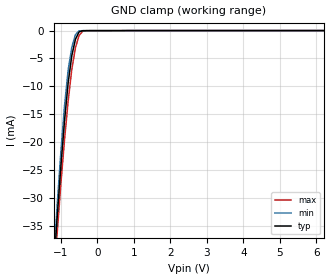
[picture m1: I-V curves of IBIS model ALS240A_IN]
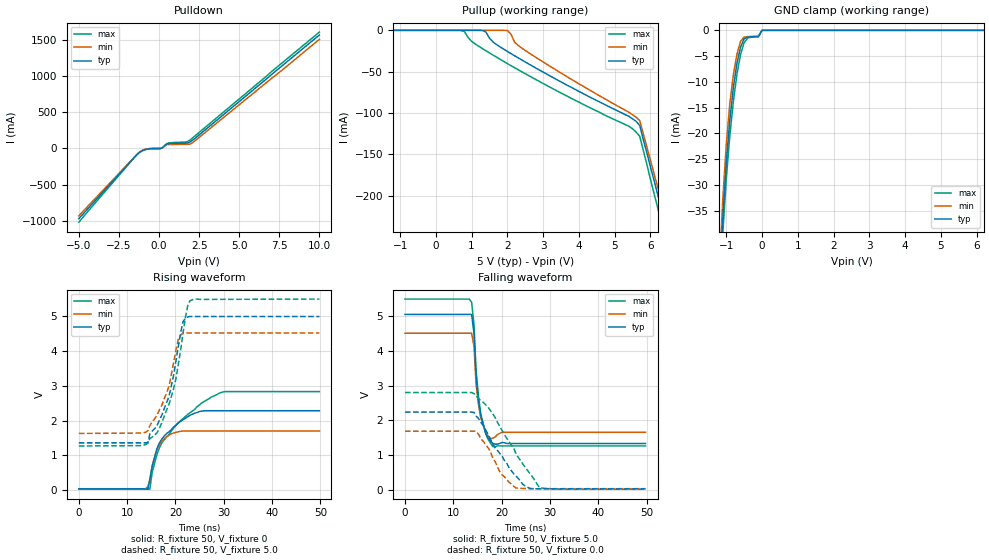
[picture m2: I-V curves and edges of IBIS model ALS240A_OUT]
| TEXAS INSTRUMENTS INCORPORATED
| Standard Linear and Logic Group
| IBIS Model of SN74ALS240A
| OCTAL BUFFERS/DRIVERS WITH 3-STATE OUTPUTS
| SOIC 20-pin (DW), SOP 20-pin (NS), SSOP 20-pin (DB), PDIP 20-pin (N) package
[IBIS Ver]   3.0
[Comment Char]  |_char
[File Name]   sn74als240a.ibs
[File Rev]   2.1
[Date]   Sept,22 2004
[Source]   Data created from Labo data at TI-SLL.
[Notes]   The following is an IBIS list for the ALS240A.
   - FILE REV HISTORY
   - 2.1 Re-Release IBIS file on 09/23/04
   - Power clamp data deleted as there is no power-clamp diode
|   Please contact sllibis@ti.com with questions and
|   comments concerning SLL IBIS models.
[Disclaimer] Property of Texas Instruments Incorporated.  Unauthorized
   reproduction and/or distribution is strictly prohibited.
   This product is protected under copyright law.
   Created 2000, (C) Copyright 2000, Texas Instruments Inc.,
   All Rights Reserved.
   UNLESS THERE IS A SIGNED, WRITTEN AGREEMENT TO THE
   CONTRARY, TEXAS INSTRUMENTS () IS PROVIDING THE IBIS
   MODELS  AND WITHOUT ANY WARRANTY, EXPRESSED OR
   IMPLIED.  TI assumes no liability for:
   1) the accuracy of the IBIS models provided to your
   company;
   2) the proper functioning of these IBIS Models in your
   design or for any resulting applications; or
   3) infringement of patents, copyrights or intellectual
   property rights resulting from your use of these IBIS
   models.
   TI provides IBIS Models as a service to our customers.
   You and your company shall not distribute, sell or give
   these models to anyone else without prior written
   permission from TI.
   TI reserves the right to make changes to our products or
   to discontinue any semiconductor product or service
   without notice, and advises our customers to obtain the
   latest version of relevant information to verify, before
   placing orders, that the information being relied on is
   current.
   Please be aware that your receipt and use of the IBIS
   information provided shall serve as acceptance of these
   terms and conditions.  If you do not accept these terms,
   you should return or destroy the IBIS models and any
   other accompanying information immediately.
|   Component ALS240A_DW
[Component]   ALS240A_DW
[Manufacturer]  Texas Instruments, Inc.
[Package]
|   typ   min   max
R_pkg   0.038   0.033   0.045
L_pkg   5.012nH   4.110nH   6.349nH
C_pkg   0.717pF   0.530pF   0.868pF
[Pin]   signal_name   model_name   R_pin   L_pin   C_pin
1   1OE_NOT   ALS240A_IN   0.042   6.336nH   0.865pF
2   1A1   ALS240A_IN   0.043   5.542nH   0.867pF
3   2Y4   ALS240A_OUT   0.034   4.714nH   0.732pF
4   1A2   ALS240A_IN   0.034   4.377nH   0.591pF
5   2Y3   ALS240A_OUT   0.036   4.130nH   0.533pF
6   1A3   ALS240A_IN   0.035   4.111nH   0.530pF
7   2Y2   ALS240A_OUT   0.034   4.284nH   0.583pF
8   1A4   ALS240A_IN   0.034   4.634nH   0.726pF
9   2Y1   ALS240A_OUT   0.040   5.518nH   0.865pF
10   GND   GND   0.043   6.349nH   0.866pF
11   2A1   ALS240A_IN   0.041   6.281nH   0.861pF
12   1Y4   ALS240A_OUT   0.045   5.561nH   0.868pF
13   2A2   ALS240A_IN   0.033   4.778nH   0.742pF
14   1Y3   ALS240A_OUT   0.035   4.414nH   0.596pF
15   2A3   ALS240A_IN   0.035   4.110nH   0.533pF
16   1Y2   ALS240A_OUT   0.036   4.130nH   0.533pF
17   2A4   ALS240A_IN   0.034   4.377nH   0.591pF
18   1Y1   ALS240A_OUT   0.034   4.714nH   0.731pF
19   2OE_NOT   ALS240A_IN   0.043   5.569nH   0.868pF
20   VCC   POWER   0.042   6.308nH   0.864pF
|   Component ALS240A_NS
[Component]   ALS240A_NS
[Manufacturer]  Texas Instruments, Inc.
[Package]
|   typ   min   max
R_pkg   0.044   0.029   0.058
L_pkg   3.666nH   2.317nH   5.115nH
C_pkg   0.548pF   0.316pF   0.725pF
[Pin]   signal_name   model_name   R_pin   L_pin   C_pin
1   1OE_NOT   ALS240A_IN   0.058   5.115nH   0.725pF
2   1A1   ALS240A_IN   0.053   4.591nH   0.724pF
3   2Y4   ALS240A_OUT   0.049   3.754nH   0.572pF
4   1A2   ALS240A_IN   0.029   2.549nH   0.388pF
5   2Y3   ALS240A_OUT   0.031   2.317nH   0.316pF
6   1A3   ALS240A_IN   0.031   2.317nH   0.316pF
7   2Y2   ALS240A_OUT   0.029   2.556nH   0.399pF
8   1A4   ALS240A_IN   0.049   3.754nH   0.579pF
9   2Y1   ALS240A_OUT   0.053   4.591nH   0.724pF
10   GND   GND   0.058   5.115nH   0.725pF
11   2A1   ALS240A_IN   0.058   5.115nH   0.725pF
12   1Y4   ALS240A_OUT   0.053   4.591nH   0.724pF
13   2A2   ALS240A_IN   0.049   3.754nH   0.579pF
14   1Y3   ALS240A_OUT   0.029   2.557nH   0.399pF
15   2A3   ALS240A_IN   0.031   2.317nH   0.316pF
16   1Y2   ALS240A_OUT   0.031   2.317nH   0.316pF
17   2A4   ALS240A_IN   0.029   2.557nH   0.399pF
18   1Y1   ALS240A_OUT   0.049   3.754nH   0.579pF
19   2OE_NOT   ALS240A_IN   0.053   4.591nH   0.724pF
20   VCC   POWER   0.058   5.115nH   0.725pF
|   Component ALS240A_DB
[Component]   ALS240A_DB
[Manufacturer]  Texas Instruments, Inc.
[Package]
|   typ   min   max
R_pkg   0.040   0.035   0.051
L_pkg   3.495nH   3.035nH   4.314nH
C_pkg   0.420pF   0.346pF   0.502pF
[Pin]   signal_name   model_name   R_pin   L_pin   C_pin
1   1OE_NOT   ALS240A_IN   0.049   4.310nH   0.502pF
2   1A1   ALS240A_IN   0.048   3.903nH   0.487pF
3   2Y4   ALS240A_OUT   0.035   3.189nH   0.396pF
4   1A2   ALS240A_IN   0.035   3.036nH   0.347pF
5   2Y3   ALS240A_OUT   0.035   3.035nH   0.367pF
6   1A3   ALS240A_IN   0.035   3.035nH   0.367pF
7   2Y2   ALS240A_OUT   0.035   3.036nH   0.347pF
8   1A4   ALS240A_IN   0.035   3.189nH   0.397pF
9   2Y1   ALS240A_OUT   0.047   3.899nH   0.488pF
10   GND   GND   0.051   4.314nH   0.500pF
11   2A1   ALS240A_IN   0.051   4.314nH   0.500pF
12   1Y4   ALS240A_OUT   0.047   3.899nH   0.488pF
13   2A2   ALS240A_IN   0.035   3.189nH   0.397pF
14   1Y3   ALS240A_OUT   0.035   3.036nH   0.346pF
15   2A3   ALS240A_IN   0.035   3.035nH   0.367pF
16   1Y2   ALS240A_OUT   0.035   3.035nH   0.367pF
17   2A4   ALS240A_IN   0.035   3.036nH   0.346pF
18   1Y1   ALS240A_OUT   0.035   3.189nH   0.397pF
19   2OE_NOT   ALS240A_IN   0.047   3.899nH   0.488pF
20   VCC   POWER   0.051   4.314nH   0.502pF
|   Component ALS240A_N
[Component]   ALS240A_N
[Manufacturer]   Texas Instruments, Inc.
[Package]
|   typ   min   max
R_pkg   4.300e-02   3.800e-02   5.000e-02
L_pkg   7.384e-09   4.680e-09   1.032e-08
C_pkg   5.100e-13   2.310e-13   8.210e-13
[Pin]   signal_name   model_name   R_pin   L_pin   C_pin
1   1OE_NOT   ALS240A_IN   4.200e-02   9.427e-09   8.100e-13
2   1A1   ALS240A_IN   4.600e-02   8.544e-09   4.560e-13
3   2Y4   ALS240A_OUT   4.800e-02   7.163e-09   4.350e-13
4   1A2   ALS240A_IN   4.000e-02   4.825e-09   2.610e-13
5   2Y3   ALS240A_OUT   4.000e-02   5.284e-09   6.480e-13
6   1A3   ALS240A_IN   4.000e-02   4.686e-09   2.320e-13
7   2Y2   ALS240A_OUT   4.000e-02   6.359e-09   4.890e-13
8   1A4   ALS240A_IN   3.800e-02   7.982e-09   4.750e-13
9   2Y1   ALS240A_OUT   4.300e-02   9.403e-09   4.750e-13
10   GND   GND   5.000e-02   1.032e-08   8.050e-13
11   2A1   ALS240A_IN   5.000e-02   1.028e-08   8.100e-13
12   1Y4   ALS240A_OUT   4.300e-02   9.383e-09   4.770e-13
13   2A2   ALS240A_IN   3.800e-02   7.978e-09   4.760e-13
14   1Y3   ALS240A_OUT   4.000e-02   6.302e-09   4.920e-13
15   2A3   ALS240A_IN   4.000e-02   4.680e-09   2.310e-13
16   1Y2   ALS240A_OUT   4.000e-02   5.284e-09   6.480e-13
17   2A4   ALS240A_IN   4.000e-02   4.822e-09   2.610e-13
18   1Y1   ALS240A_OUT   4.700e-02   7.118e-09   4.390e-13
19   2OE_NOT   ALS240A_IN   4.600e-02   8.492e-09   4.610e-13
20   VCC   POWER   4.300e-02   9.348e-09   8.210e-13
| Models and submodels in the file (2): ALS240A_IN (Input), ALS240A_OUT (3-state)
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|   Model ALS240A_IN
[Model]   ALS240A_IN
Model_type  Input
Polarity   Non-Inverting
Vinl = 0.8
Vinh = 2.0
| variable   typ   min   max
C_comp   1.33pf   1.00pf   1.66pf
[Temperature Range]   25   0   70
[Voltage Range]   5.0   4.5   5.5
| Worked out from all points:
|   GND clamp passes 1 mA (typ) near -0.56 V on its own axis
[GND Clamp]
|   Voltage   I(typ)   I(min)   I(max)
-5V       -461mA     -433mA     -495mA
-1.2V     -43.3mA    -41.8mA    -45.3mA
-1.1V     -33.5mA    -31.3mA    -36.4mA
-1V       -24.5mA    -21.9mA    -27.6mA
-900mV    -16.3mA    -13.6mA    -19.7mA
-800mV    -9.41mA    -7.13mA    -12.7mA
-700mV    -4.51mA    -3.02mA    -6.98mA
-600mV    -1.57mA    -736uA     -3.07mA
-500mV    -228uA     -51uA      -886uA
-400mV    -23.3uA    -17.2uA    -118uA
-300mV    -14.7uA    -15.9uA    -18.4uA
10V       1.67nA     128pA      258pA
|   Model ALS240A_OUT
[Model]   ALS240A_OUT
Model_type  3-state
Polarity   Inverting
Enable   Active-Low
Vmeas = 1.3v
Cref = 0pf
| variable   typ   min   max
C_comp   5.8pf   4.35pf   7.25pf
[Temperature Range]   25   0   70
[Voltage Range]   5.0   4.5   5.5
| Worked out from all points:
|   slope of the pulldown table from 0 to 0.75 V, typ, clamps not added: 10.6 ohm
|   rising waveform, R_fixture 50, V_fixture 0: 20-80 % time 4.86ns typ, 2.19ns min, 8.17ns max; typ from 0.044 V to 2.28 V
|   falling waveform, R_fixture 50, V_fixture 5.0: 20-80 % time 1.44ns typ, 1.13ns min, 1.5ns max; typ from 5.04 V to 1.34 V
|   rising waveform, R_fixture 50, V_fixture 5.0: 20-80 % time 3.82ns typ, 3.64ns min, 4.07ns max; typ from 1.36 V to 4.98 V
|   falling waveform, R_fixture 50, V_fixture 0.0: 20-80 % time 6.06ns typ, 4.24ns min, 7.4ns max; typ from 2.24 V to 0.04 V
[Pulldown]
|   Voltage   I(typ)   I(min)   I(max)
-5V       -971mA     -932mA     -1.02A
-1.3V     -68.5mA    -66mA      -70.7mA
-1.1V     -36.8mA    -33.2mA    -39.8mA
-800mV    -11mA      -8.54mA    -13.7mA
100mV     -270uA     -649uA     281uA
200mV     7.68mA     5.22mA     9.57mA
500mV     63.2mA     53.1mA     68.2mA
1.7V      74.2mA     57.1mA     90.5mA
2V        99.7mA     66.7mA     127mA
10V       1.57A      1.51A      1.61A
[Pullup]
|   Voltage   I(typ)   I(min)   I(max)
-5V       510pA      14.2pA     2.91nA
700mV     508pA      12.2pA     -71.8uA
1.4V      -2.04mA    12.2pA     -24.7mA
1.6V      -14.2mA    -11.3pA    -30mA
2V        -25.5mA    -258uA     -40.2mA
2.4V      -35.7mA    -21.4mA    -50mA
5.4V      -104mA     -99.1mA    -116mA
5.7V      -115mA     -109mA     -128mA
6.3V      -215mA     -204mA     -232mA
6.4V      -231mA     -220mA     -249mA
6.5V      -248mA     -236mA     -266mA
10V       -827mA     -792mA     -872mA
[GND Clamp]
|   Voltage   I(typ)   I(min)   I(max)
-5V       -971mA     -932mA     -1.02A
-1.2V     -51mA      -47.7mA    -53.7mA
-1.1V     -36.8mA    -33.2mA    -39.8mA
-1V       -25.7mA    -22.2mA    -28.9mA
-900mV    -17.4mA    -14.2mA    -20.4mA
-800mV    -11mA      -8.54mA    -13.7mA
-700mV    -6.35mA    -4.58mA    -8.47mA
-600mV    -3.23mA    -2.14mA    -4.67mA
-500mV    -1.65mA    -1.31mA    -2.37mA
-100mV    -1.19mA    -1.13mA    -1.26mA
0V        1.12uA     1.09uA     1.13uA
10V       1.12uA     1.09uA     1.13uA
[Ramp]
| variable   typ   min   max
dV/dt_r   1.37E+00/5.19E-09   1.18E+00/4.47E-09   1.52E+00/6.82E-09
dV/dt_f   2.16E+00/1.23E-09   1.74E+00/1.12E-09   2.52E+00/1.45E-09
R_load = 50
[Rising Waveform]
R_fixture = 50
V_fixture = 0
|   Time   V(typ)   V(min)   V(max)
0s        43.7mV     45.7mV     34.5mV
14.3ns    39mV       104mV      34.6mV
14.7ns    320mV      282mV      33.2mV
15.2ns    690mV      714mV      522mV
16.2ns    1.2V       1.18V      1.04V
18.2ns    1.63V      1.54V      1.53V
20.6ns    1.93V      1.68V      1.94V
24ns      2.21V      1.7V       2.32V
29.4ns    2.28V      1.7V       2.8V
49.8ns    2.28V      1.7V       2.83V
[Falling Waveform]
R_fixture = 50
V_fixture = 5.0
V_fixture_min = 4.5
V_fixture_max = 5.5
|   Time   V(typ)   V(min)   V(max)
0s        5.04V      4.5V       5.48V
13.8ns    5.04V      4.5V       5.39V
14.3ns    4.48V      4.11V      4.73V
14.7ns    3.3V       3.07V      3.46V
15.2ns    2.58V      2.47V      2.71V
15.7ns    2.13V      2.07V      2.18V
16.7ns    1.64V      1.68V      1.63V
18.2ns    1.34V      1.49V      1.25V
20.1ns    1.37V      1.66V      1.27V
49.8ns    1.34V      1.66V      1.27V
[Rising Waveform]
R_fixture = 50
V_fixture = 5.0
V_fixture_min = 4.5
V_fixture_max = 5.5
|   Time   V(typ)   V(min)   V(max)
0s        1.36V      1.63V      1.27V
14.3ns    1.37V      1.71V      1.35V
14.7ns    1.61V      1.85V      1.48V
16.2ns    1.86V      2.16V      1.65V
18.7ns    2.71V      3V         2.48V
20.6ns    4.12V      4.33V      3.61V
21.6ns    4.84V      4.5V       4.53V
22.6ns    4.97V      4.51V      5.32V
23ns      4.98V      4.51V      5.43V
49.8ns    4.98V      4.51V      5.48V
[Falling Waveform]
R_fixture = 50
V_fixture = 0.0
|   Time   V(typ)   V(min)   V(max)
0s        2.24V      1.69V      2.8V
14.3ns    2.23V      1.69V      2.77V
15.2ns    2.06V      1.61V      2.63V
17.2ns    1.6V       1.22V      2.38V
18.2ns    1.32V      917mV      2.19V
20.1ns    980mV      443mV      1.71V
22.6ns    458mV      99.1mV     1.18V
25ns      111mV      47.6mV     643mV
27.9ns    40.2mV     44mV       71.2mV
49.8ns    40.2mV     44mV       29.8mV
